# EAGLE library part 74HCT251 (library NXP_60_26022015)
8-input multiplexer; 3-state The 74HC251; 74HCT251 is an 8-bit multiplexer with eight binary inputs (I0 to I7), three select inputs (S0 to S2) and an output enable input (OE). The select inputs select one of the eight binary inputs and route it to the complementary outputs (Y and Y). A HIGH on OE causes the outputs to assume a high-impedance OFF-state. Inputs include clamp diodes that enable the use of current limiting resistors to interface inputs to voltages in excess of VCC. AAL Eindhoven MK
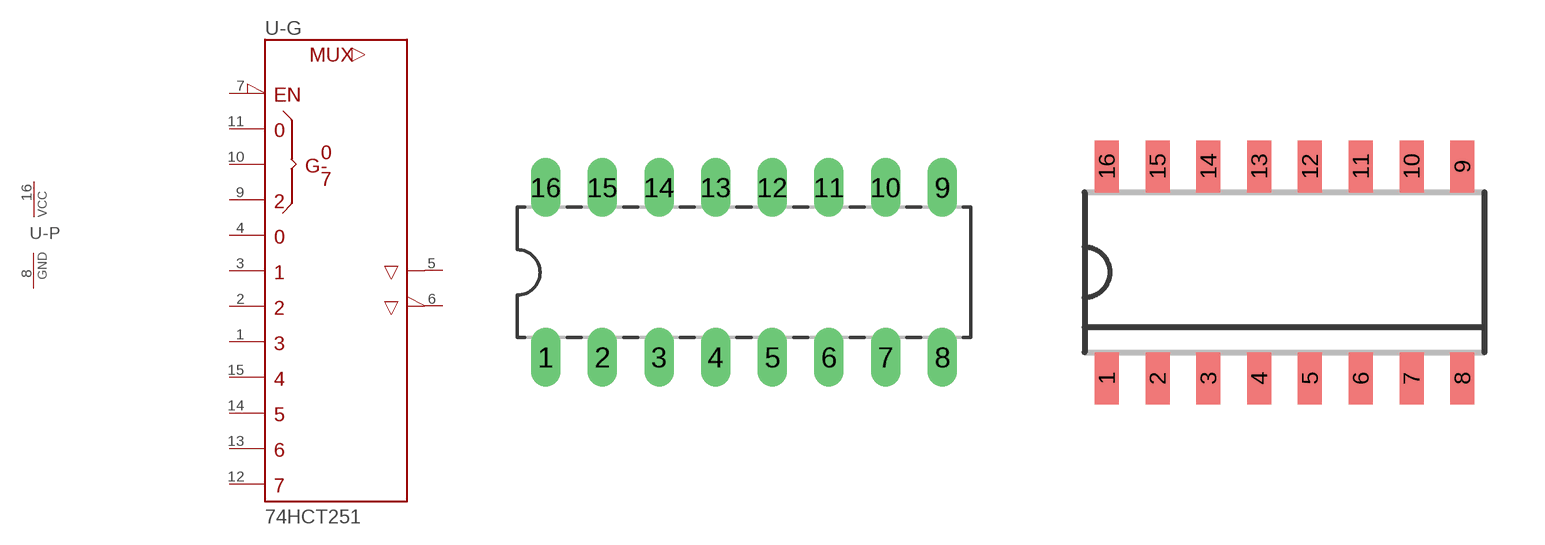
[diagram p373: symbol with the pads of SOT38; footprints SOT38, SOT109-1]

Designator prefix U; gates -G=251 -P=PWRN

## 74HCT251N  [SOT38]
1  -G:D3  in
2  -G:D2  in
3  -G:D1  in
4  -G:D0  in
5  -G:Y  hiz
6  -G:W  hiz
7  -G:!G  in
8  -P:GND  pwr
9  -G:C  in
10  -G:B  in
11  -G:A  in
12  -G:D7  in
13  -G:D6  in
14  -G:D5  in
15  -G:D4  in
16  -P:VCC  pwr

## 74HCT251D  [SOT109-1]
Pads as for SOT38

## 74HCT251DP  [SOT338]
Pads as for SOT38

## 74HCT251PW  [SOT403-1]
Pads as for SOT38

## Footprint SOT38 (pad centres in mm)
Dual In Line Package
drill 0.813 long: 1 -8.89,-3.81; 2 -6.35,-3.81; 3 -3.81,-3.81; 4 -1.27,-3.81; 5 1.27,-3.81; 6 3.81,-3.81; 7 6.35,-3.81; 8 8.89,-3.81; 9 8.89,3.81; 10 6.35,3.81; 11 3.81,3.81; 12 1.27,3.81; 13 -1.27,3.81; 14 -3.81,3.81; 15 -6.35,3.81; 16 -8.89,3.81

## Footprint SOT109-1 (pad centres in mm)
SOT109-1 SO16: plastic small outline package; 16 leads; body width 3.9 mm JEDEC: MS-012 IEC: 076E07
smd 0.6 x 1.3: 1 -4.445,-2.65; 2 -3.175,-2.65; 3 -1.905,-2.65; 4 -0.635,-2.65; 5 0.635,-2.65; 6 1.905,-2.65; 7 3.175,-2.65; 8 4.445,-2.65; 9 4.445,2.65; 10 3.175,2.65; 11 1.905,2.65; 12 0.635,2.65; 13 -0.635,2.65; 14 -1.905,2.65; 15 -3.175,2.65; 16 -4.445,2.65

## Footprint SOT338 (pad centres in mm)
SOT338 SSOP16: plastic shrink small outline package; 16 leads; body width 5.3 mm JEDEC: MO-150 IEC: --
smd 0.4 x 1.2: 1 -2.275,-3.45; 2 -1.625,-3.45; 3 -0.975,-3.45; 4 -0.325,-3.45; 5 0.325,-3.45; 6 0.975,-3.45; 7 1.625,-3.45; 8 2.275,-3.45; 9 2.275,3.45; 10 1.625,3.45; 11 0.975,3.45; 12 0.325,3.45; 13 -0.325,3.45; 14 -0.975,3.45; 15 -1.625,3.45; 16 -2.275,3.45

## Footprint SOT403-1 (pad centres in mm)
SOT403-1 TSSOP16: plastic thin shrink small outline package; 16 leads; body width 4.4 mm JEDEC: MO-153 IEC: ---
smd 0.6 x 1.35: 1 -2.375,-2.925; 8 2.375,-2.925; 9 2.375,2.925; 16 -2.375,2.925
smd 0.4 x 1.35: 2 -1.625,-2.925; 3 -0.975,-2.925; 4 -0.325,-2.925; 5 0.325,-2.925; 6 0.975,-2.925; 7 1.625,-2.925; 10 1.625,2.925; 11 0.975,2.925; 12 0.325,2.925; 13 -0.325,2.925; 14 -0.975,2.925; 15 -1.625,2.925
